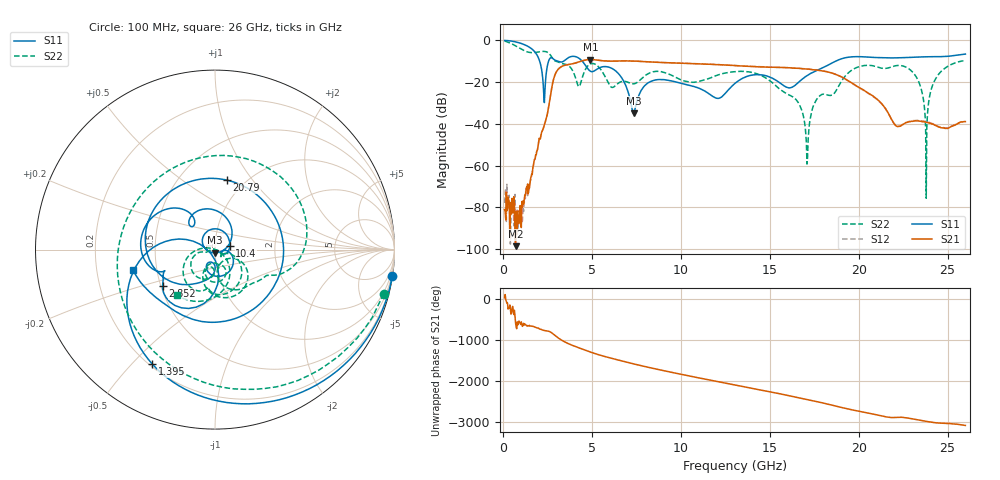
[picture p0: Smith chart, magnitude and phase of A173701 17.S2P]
!  2-Port S-parameters saved by WinCal
! VAR MeasName=S-Parameters (CALIBRATED_DATA) read from VNA (N5245A)
! VAR MeasDate=2017-6-7 10:29:30
! VAR NAME=A173701 17
! VAR FILENAME=A173701 17.S2P
! VAR DATE=2017-6-7 10:29:30
! VAR PHYS_PORTS=1,2
# Hz S DB R 50
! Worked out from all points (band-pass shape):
!   801 points, 100 MHz to 26 GHz, reference 50 ohm
!   highest |S21| = -9.15 dB at 4.924 GHz (marker M1); lowest = -98.7 dB at 715.1 MHz (marker M2)
!   |S21| within 3 dB of the highest: 3.399 GHz to 13.21 GHz (9.808 GHz wide, 118 % of centre); 13.21994 GHz to 13.25586 GHz (35.92 MHz wide, 0.271 % of centre)
!   lowest |S11| = -35.0 dB at 7.352 GHz (marker M3), VSWR 1.04, Z = 49.9 - j1.77 ohm
!   |S11| at or under -10 dB: 2.072 GHz to 2.57 GHz (497.9 MHz wide, 21.5 % of centre); 3.111 GHz to 3.406 GHz (295.3 MHz wide, 9.06 % of centre); 4.469 GHz to 18.69 GHz (14.22 GHz wide, 123 % of centre)
!   |S22| runs from -75.7 to -0.2 dB; largest |S21 - S12| = 0.0038
!   S11 on the Smith chart (normalised r, x): 100 MHz: 0, -13; 1.395 GHz: 0.21, -0.57; 2.852 GHz: 0.51, -0.24; 10.4 GHz: 1.18, +0.05; 20.79 GHz: 0.83, +0.76; 26 GHz: 0.36, -0.11
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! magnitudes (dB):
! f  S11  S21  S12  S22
! 100 MHz  0.0  -81.1  -77.9  -0.2
! 715.1 MHz  -0.7  -98.7  -84.0  -2.6
! 1.395 GHz  -2.8  -68.8  -74.4  -5.5
! 2.301 GHz  -26.0  -41.6  -41.5  -5.3
! 2.852 GHz  -9.0  -18.6  -18.6  -9.2
! 4.438 GHz  -9.7  -9.8  -9.9  -18.6
! 4.924 GHz  -14.8  -9.1  -9.2  -11.3
! 6.381 GHz  -14.9  -9.9  -9.9  -21.3
! 7.352 GHz  -35.0  -9.9  -9.9  -20.8
! 8.744 GHz  -18.8  -10.5  -10.5  -14.8
! 10.4 GHz  -21.4  -11.0  -11.0  -19.8
! 12.08 GHz  -27.8  -11.6  -11.6  -16.6
! 13.05 GHz  -20.6  -12.0  -12.1  -15.0
! 16.42 GHz  -21.6  -13.3  -13.2  -27.9
! 17.1 GHz  -16.9  -13.7  -13.7  -59.3
! 17.39 GHz  -15.4  -14.0  -13.9  -33.2
! 20.79 GHz  -8.1  -26.5  -26.8  -12.1
! 21.69 GHz  -8.4  -35.3  -35.3  -13.1
! 23.18 GHz  -8.0  -38.5  -38.4  -16.8
! 23.8 GHz  -7.8  -39.3  -39.0  -75.7
! 24.38 GHz  -7.8  -40.9  -40.9  -17.6
! 26 GHz  -6.5  -38.9  -38.9  -9.7
